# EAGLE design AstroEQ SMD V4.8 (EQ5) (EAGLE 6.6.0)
REVISION: V4.8
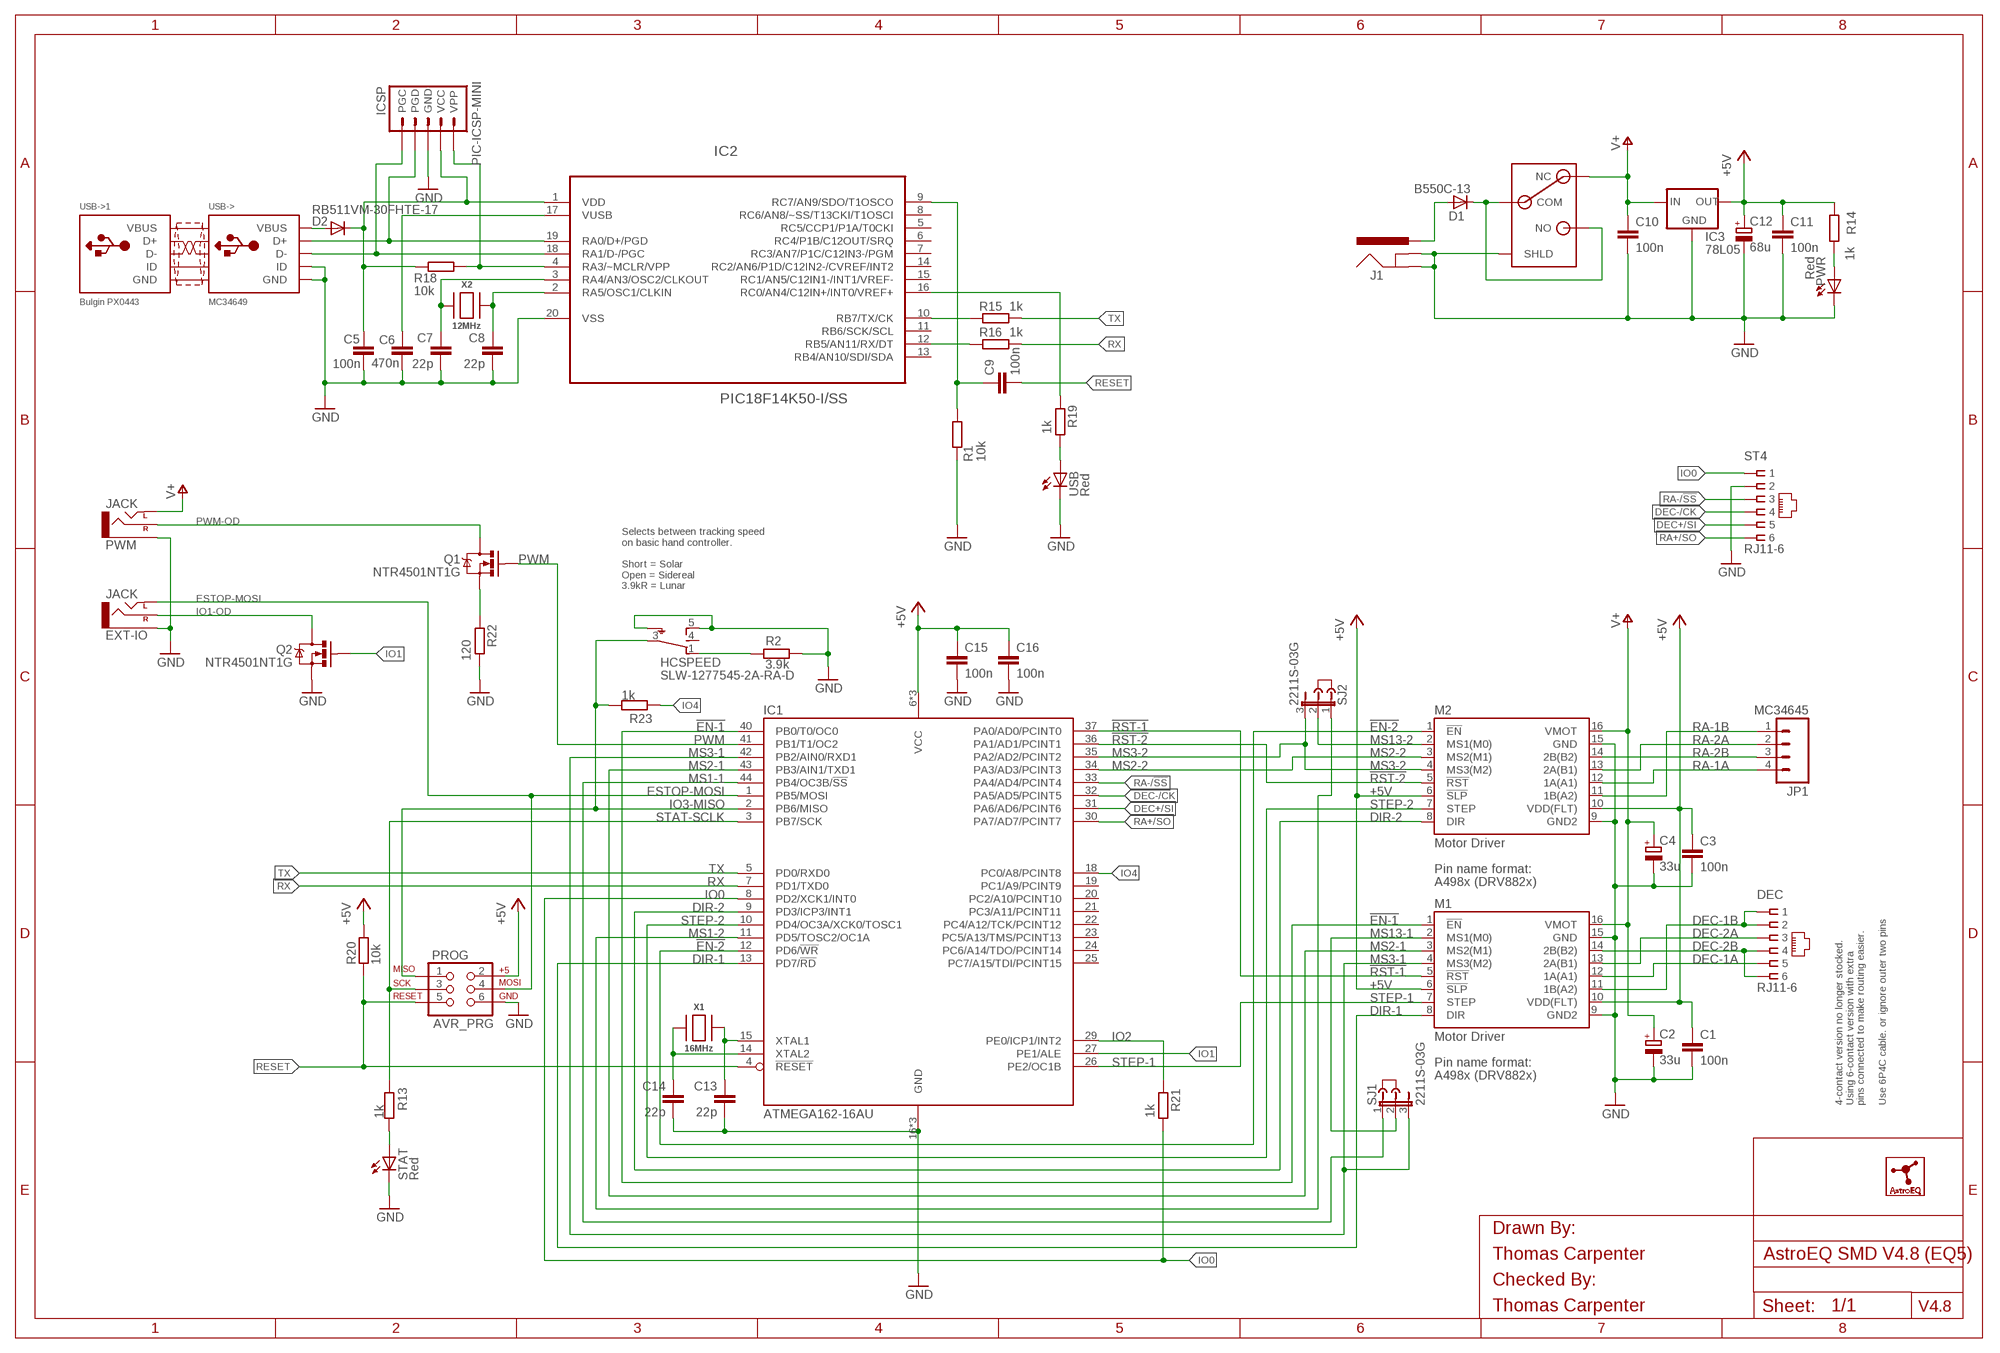
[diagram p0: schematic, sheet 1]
FRAME1 (A3L-LOC): CHECKED_BY: Thomas Carpenter; DRAWN_BY: Thomas Carpenter
USB->1 (USB-PANEL): MF: BULGIN; MPN: PX0443; OC_FARNELL: 1229685

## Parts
C1  100n  C-EUC0603  [C0603]
C2  33u  CPOL-EUSMCC  [SMC_C]
C3  100n  C-EUC0603  [C0603]
C4  33u  CPOL-EUSMCC  [SMC_C]
C5  100n  C-EUC0603  [C0603]
C6  470n  C-EUC0603  [C0603]
C7  22p  C-EUC0603  [C0603]
C8  22p  C-EUC0603  [C0603]
C9  100n  C-EUC0603  [C0603]
C10  100n  C-EUC0603  [C0603]
C11  100n  C-EUC0603  [C0603]
C12  68u  CPOL-EUSMCC  [SMC_C]
C13  22p  C-EUC0603  [C0603]
C14  22p  C-EUC0603  [C0603]
C15  100n  C-EUC0603  [C0603]
C16  100n  C-EUC0603  [C0603]
D1  B550C-13  DIODE-SMC  [SMC]
D2  RB511VM-30FHTE-17  DIODESOD  [SOD-323]
DEC  RJ11-6  RJ11-2L-B  [RJ11-NO_SHIELD]
EXT-IO  JACK  AUDIO-JACKVERT  [AUDIO-JACK-3.5MM-VERT]
HCSPEED  SLW-1277545-2A-RA-D  [SLW-127]
IC1  ATMEGA162-16AU  [TQFP44]
IC2  PIC18F14K50-I/SS  [SS20]
IC3  78L05  78LXXSOT-23  [SOT23]
ICSP  PIC-ICSP-MINI  [PIC-ICSP-MINI]
J1  POWER_JACKPANEL  [POWER_JACK_PANEL]
J2  DNI  JUMPER  [JUMP]
J3  DNI  JUMPER  [JUMP]
JP1  MC34645  M04POLAR  [MOLEX-1X4]
LOGO1  ASTROEQ5MM  [ASTROEQ-SMALL]
M1  Motor Driver  A4983CARRIER  [DIP16-W]
M2  Motor Driver  A4983CARRIER  [DIP16-W]
PROG  AVR_PRG  AVR_SPI_PRG_6PTH  [2X3]
PWM  JACK  AUDIO-JACKVERT  [AUDIO-JACK-3.5MM-VERT]
PWR  Red  LED3MM  [LED3MM]
PWR-SW  SWITCH  [SPST]
Q1  NTR4501NT1G  MOSFET-NCHANNELSMD  [SOT23-3]
Q2  NTR4501NT1G  MOSFET-NCHANNELSMD  [SOT23-3]
R1  10k  R-EU_R0603  [R0603]
R2  3.9k  R-EU_R0603  [R0603]
R13  1k  R-EU_R0603  [R0603]
R14  1k  R-EU_R0603  [R0603]
R15  1k  R-EU_R0603  [R0603]
R16  1k  R-EU_R0603  [R0603]
R18  10k  R-EU_R0603  [R0603]
R19  1k  R-EU_R0603  [R0603]
R20  10k  R-EU_R0603  [R0603]
R21  1k  R-EU_R0603  [R0603]
R22  120  R-EU_R0805  [R0805]
R23  1k  R-EU_R0603  [R0603]
SJ1  2211S-03G  JP2E  [JP2]
SJ2  2211S-03G  JP2E  [JP2]
ST4  RJ11-6  RJ11-2L-B  [RJ11-NO_SHIELD]
STAT  Red  LED3MM  [LED3MM]
USB  Red  LED3MM  [LED3MM]
USB->  MC34649  USBBULGINWIRE  [22-23-2051]
X1  16MHz  XTALNX5032  [NX5032]
X2  12MHz  XTALNX5032  [NX5032]

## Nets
!EN-1: IC1.40(PB0/T0/OC0) M1.1(!EN)
!EN-2: IC1.12(PD6/!WR) M2.1(!EN)
!RST-1: IC1.37(PA0/AD0/PCINT0) M1.5(!RST)
!RST-2: IC1.36(PA1/AD1/PCINT1) M2.5(!RST)
+5V: C1.1 C3.1 C11.1 C12.+ C15.1 C16.1 IC1.6(VCC) IC1.17(VCC) IC1.38(VCC) IC3.1(OUT) M1.6(!SLP) M1.10(VDD(FLT)) M2.6(!SLP) M2.10(VDD(FLT)) PROG.2 R14.1 R20.2
AVROSC1: C13.1 IC1.15(XTAL1) X1.1
AVROSC2: C14.1 IC1.14(XTAL2) X1.2
D_N [usbdat]: IC2.18(RA1/D-/PGC) ICSP.5(PGC) USB->.2(D-)
D_P [usbdat]: IC2.19(RA0/D+/PGD) ICSP.4(PGD) USB->.3(D+)
DEC+/SI: IC1.31(PA6/AD6/PCINT6) ST4.5
DEC-1A: DEC.5 M1.12(1A(A1))
DEC-1B: DEC.1 DEC.2 M1.11(1B(A2))
DEC-2A: DEC.3 M1.13(2A(B1))
DEC-2B: DEC.4 DEC.6 M1.14(2B(B2))
DEC-/CK: IC1.32(PA5/AD5/PCINT5) ST4.4
DIR-1: IC1.13(PD7/!RD) M1.8(DIR)
DIR-2: IC1.9(PD3/ICP3/INT1) M2.8(DIR)
DTR: C9.1 IC2.9(RC7/AN9/SDO/T1OSCO) R1.1
ESTOP-MOSI: EXT-IO.2(LEFT) IC1.1(PB5/MOSI) PROG.4
GND: C1.2 C2.- C3.2 C4.- C5.2 C6.1 C7.2 C8.2 C10.2 C11.2 C12.- C13.2 C14.2 C15.2 C16.2 EXT-IO.1(SLEEVE) HCSPEED.5(O) HCSPEED.S1(SH) HCSPEED.S2(SH) IC1.16(GND) IC1.28(GND) IC1.39(GND) IC2.20(VSS) IC3.3(GND) ICSP.3(GND) J1.SHUNT(GNDBREAK) J1.SLEEVE(GND) M1.9(GND2) M1.15(GND) M2.9(GND2) M2.15(GND) PROG.6 PWM.1(SLEEVE) PWR-SW.S1(SHLD) PWR-SW.S2(SHLD) PWR-SW.S3(SHLD) PWR-SW.S4(SHLD) PWR.K(C) Q2.2(S) R1.2 R2.2 R22.1 ST4.2 STAT.K(C) USB->.4(GND) USB->.5(ID) USB.K(C)
IO0: IC1.8(PD2/XCK1/INT0) R21.1 ST4.1
IO1: IC1.27(PE1/ALE) Q2.1(G)
IO1-OD: EXT-IO.3(RIGHT) Q2.3(D)
IO2: IC1.29(PE0/ICP1/INT2) R21.2
IO3-MISO: HCSPEED.3(P) IC1.2(PB6/MISO) PROG.1 R23.2
IO4: IC1.18(PC0/A8/PCINT8) R23.1
MCLR: IC2.4(RA3/~MCLR/VPP) ICSP.1(VPP) R18.1
MS1-1: IC1.44(PB4/OC3B/!SS) SJ1.1
MS1-2: IC1.11(PD5/TOSC2/OC1A) SJ2.1
MS2-1: IC1.43(PB3/AIN1/TXD1) M1.3(MS2(M1))
MS2-2: IC1.34(PA3/AD3/PCINT3) M2.3(MS2(M1))
MS3-1: IC1.42(PB2/AIN0/RXD1) M1.4(MS3(M2)) SJ1.3
MS3-2: IC1.35(PA2/AD2/PCINT2) M2.4(MS3(M2)) SJ2.3
MS13-1: M1.2(MS1(M0)) SJ1.2
MS13-2: M2.2(MS1(M0)) SJ2.2
N$1: HCSPEED.1(S) R2.1
PWM: IC1.41(PB1/T1/OC2) Q1.1(G)
PWM-OD: PWM.3(RIGHT) Q1.3(D)
PWM-RES: Q1.2(S) R22.2
PWRLED: PWR.A R14.2
RA+/SO: IC1.30(PA7/AD7/PCINT7) ST4.6
RA-1A: JP1.4 M2.12(1A(A1))
RA-1B: JP1.1 M2.11(1B(A2))
RA-2A: JP1.2 M2.13(2A(B1))
RA-2B: JP1.3 M2.14(2B(B2))
RA-/!SS: IC1.33(PA4/AD4/PCINT4) ST4.3
RESET: C9.2 IC1.4(!RESET) PROG.5 R20.1
RX: IC1.7(PD1/TXD0) R16.1
RX(USB): IC2.12(RB5/AN11/RX/DT) R16.2
STAT-SCLK: IC1.3(PB7/SCK) PROG.3 R13.1
STATLED: R13.2 STAT.A
STEP-1: IC1.26(PE2/OC1B) M1.7(STEP)
STEP-2: IC1.10(PD4/OC3A/XCK0/TOSC1) M2.7(STEP)
SWITCH: D1.C PWR-SW.COM PWR-SW.NO
TX: IC1.5(PD0/RXD0) R15.1
TX(USB): IC2.10(RB7/TX/CK) R15.2
USBLED: R19.1 USB.A
USBOSC1: C8.1 IC2.2(RA5/OSC1/CLKIN) X2.2
USBOSC2: C7.1 IC2.3(RA4/AN3/OSC2/CLKOUT) X2.1
USBSTAT: IC2.16(RC0/AN4/C12IN+/INT0/VREF+) R19.2
V+: C2.+ C4.+ C10.1 IC3.2(IN) M1.16(VMOT) M2.16(VMOT) PWM.2(LEFT) PWR-SW.NC
VBUS: D2.2(A) USB->.1(VBUS)
VIN: D1.A J1.CENTRE(PWR)
VPIC: C5.1 D2.1(C) IC2.1(VDD) ICSP.2(VCC) R18.2
VUSB: C6.2 IC2.17(VUSB)
Unconnected: HCSPEED.4(M) IC1.19(PC1/A9/PCINT9) IC1.20(PC2/A10/PCINT10) IC1.21(PC3/A11/PCINT11) IC1.22(PC4/A12/TCK/PCINT12) IC1.23(PC5/A13/TMS/PCINT13) IC1.24(PC6/A14/TDO/PCINT14) IC1.25(PC7/A15/TDI/PCINT15) IC2.5(RC5/CCP1/P1A/T0CKI) IC2.6(RC4/P1B/C12OUT/SRQ) IC2.7(RC3/AN7/P1C/C12IN3-/PGM) IC2.8(RC6/AN8/~SS/T13CKI/T1OSCI) IC2.11(RB6/SCK/SCL) IC2.13(RB4/AN10/SDI/SDA) IC2.14(RC2/AN6/P1D/C12IN2-/CVREF/INT2) IC2.15(RC1/AN5/C12IN1-/INT1/VREF-)

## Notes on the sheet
- Selects between tracking speed
  on basic hand controller.
  
  Short = Solar
  Open = Sidereal
  3.9kR = Lunar
- 4-contact version no longer stocked.
  Using 6-contact version with extra
  pins connected to make routing easier.
  
  Use 6P4C cable. or ignore outer two pins

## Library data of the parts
C1 C3 C5 C9-C11 C15 C16 = rcl:C-EU: CAPACITOR, European symbol; MF: MULTICOMP; MPN: MC0603F104Z250CT; OC_FARNELL: 1759038
C2 C4 = rcl:CPOL-EU: POLARIZED CAPACITOR, European symbol; MF: KEMET; MPN: T491C336K025AT; OC_FARNELL: 1793896
C6 = rcl:C-EU: CAPACITOR, European symbol; MF: MULTICOMP; MPN: MC0603F474Z160CT; OC_FARNELL: 1759021
C7 C8 C13 C14 = rcl:C-EU: CAPACITOR, European symbol; MF: MULTICOMP; MPN: MC0603N220J500CT; OC_FARNELL: 1759057
C12 = rcl:CPOL-EU: POLARIZED CAPACITOR, European symbol; MF: AVX; MPN: TPSC686K016R0125; OC_FARNELL: 1658976
D1 = diode:DIODE-: DIODE; MF: DIODES INC.; MPN: B550C-13-F; OC_FARNELL: 1858608
D2 = SparkFun:DIODE: Diode; MF: ROHM; MPN: RB511VM-30FHTE-17; OC_FARNELL: 2581544
DEC ST4 = con-tycoelectronics:RJ11: CORCOM Modular RJ Jacks No Shield Source: www.tycoelectronics.com .. ENG_DS_1654001_1099_RJ_L_0507.pdf; MF: MOLEX; MPN: 95503-2661; OC_FARNELL: 1620210
EXT-IO PWM = SparkFun:AUDIO-JACK: 3.5mm Audio Jack Simple 3.5mm common PCB mount audio jack. SKU: PRT-08032; MANUFACTURER: LUMBERG; MF: LUMBERG; MPN: 1502 01; OC_FARNELL: 1243242
HCSPEED = switch:SLW-127
IC1 = atmel:ATMEGA162: 8-bit RISC MICROCONTROLLER 16K Bytes internal flash program memory 1K Bytes internal SRAM Upto 64K Bytes optional external memory space 512 Bytes EEPROM Two 8-bit timers Two 16-bit timers Dual programmable serial USARTs Master/Slave serial SPI interface Source: ATMEGA162_DIP40.lbr; MF: ATMEL; MPN: ATMEGA162-16AU; OC_FARNELL: 9171150
IC2 = microchip:PIC18F14K50: USB Flash Microcontrollers; MF: MICROCHIP
IC3 = v-reg:78LXX: VOLTAGE REGULATOR; MF: TAIWAN SEMICONDUCTOR; MPN: TS78L05CX RFG; OC_FARNELL: 1476698
ICSP = SparkFun:PIC-ICSP-MINI: PIC-ICSP-Mini Miniature 5-pin connection for temporary programming of PICs. Use this device in your design to save space. Program the PIC with this adapter Spark Fun Electronics SKU : BOB-00194; OC_FARNELL: unknown
J1 = SparkFun:POWER_JACK: Power Jack This is the standard 5.5mm barrel jack for power. The PTH is the most common, proven, reliable, footprint. All others are experimental. The Slot footprint only works if the mill layer is transmitted to the PCB fab house so be warned. Spark Fun Electronics SKU : PRT-00119. Mating wall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; MF: SWITCHCRAFT; MPN: PCL712AS; OC_FARNELL: 1871167
J2 J3 = jumper:JUMPER: JUMPER header; MF: 3M; MPN: 969102-0000-DA; OC_FARNELL: 2579814
JP1 = SparkFun:M04: Header 4 Standard 4-pin 0.1" header. Use with straight break away headers (SKU : PRT-00116), right angle break away headers (PRT-00553), swiss pins (PRT-00743), machine pins (PRT-00117), and female headers (PRT-00115). Molex polarized connector foot print use with SKU : PRT-08231 with associated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; MF: MULTICOMP; MPN: MC34645; OC_FARNELL: 1675775
LOGO1 = AstroEQTooth:ASTROEQ; OC_FARNELL: unknown
M1 M2 = A4983Carrier:A4983CARRIER; MF: SAMTEC; MPN: CES-116-01-T-S; OC_FARNELL: 1667522
PROG = SparkFun:AVR_SPI_PRG_6: AVR ISP 6 Pin This is the reduced ISP connector for AVR programming. Common on Arduino. This footprint will take up less PCB space and can be used with a 10-pin to 6-pin adapter such as SKU: BOB-08508; MF: AMP - TE CONNECTIVITY; MPN: 826632-3; OC_FARNELL: 3418492
PWR STAT USB = led:LED: LED; MF: KINGBRIGHT; MPN: L-424HDT; OC_FARNELL: 1142499
PWR-SW = con-tycoelectronics:SWITCH; MF: TE CONNECTIVITY; MPN: AE101J1V3B004; OC_FARNELL: 1813654
Q1 Q2 = SparkFun:MOSFET-NCHANNEL; MF: ON SEMICONDUCTOR; MPN: NTR4501NT1G; OC_FARNELL: 1431305
R1 R18 R20 = rcl:R-EU_: RESISTOR, European symbol; MF: MULTICOMP; MPN: MCWR06X1002FTL; OC_FARNELL: 2447230
R2 R13-R16 R19 R21 R23 = rcl:R-EU_: RESISTOR, European symbol; MF: MULTICOMP; MPN: MCWR06X1001FTL; OC_FARNELL: 2447272
R22 = rcl:R-EU_: RESISTOR, European symbol; MF: MULTICOMP; MPN: MCWR08X1200FTL; OC_FARNELL: 2447561
SJ1 SJ2 = jumper:JP2E: JUMPER; MF: MULTICOMP; MPN: 2211S-03G; OC_FARNELL: 1593412
USB-> = adafruit:USB: USB Connectors USBMINIB - Surface Mount Female Mini-B USB Connector 4UConnector: 06564 By microbuilder.eu Thru-hole RA Female Mini-B USB Connector 4UConnector: 18732 By ladyada.net; MF: MULTICOMP; MPN: MC34647; OC_FARNELL: 1675776
X1 = adafruit:XTAL: Low cost SMT crystals, no capacitors included; MF: TXC; MPN: 7A-16.000MAAJ-T; OC_FARNELL: 1841946
X2 = adafruit:XTAL: Low cost SMT crystals, no capacitors included; MF: TXC; MPN: 7A-12.000MAAJ-T; OC_FARNELL: 1841940

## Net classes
1 power: width 0.61 mm, drill 0.711 mm, clearance 0.203 mm
2 gnd: width 0.305 mm, drill 0.711 mm, clearance 0.203 mm
3 usbvcc: width 0.508 mm, drill 0.711 mm, clearance 0.203 mm
4 usbdat: width 0.406 mm, clearance 0.152 mm

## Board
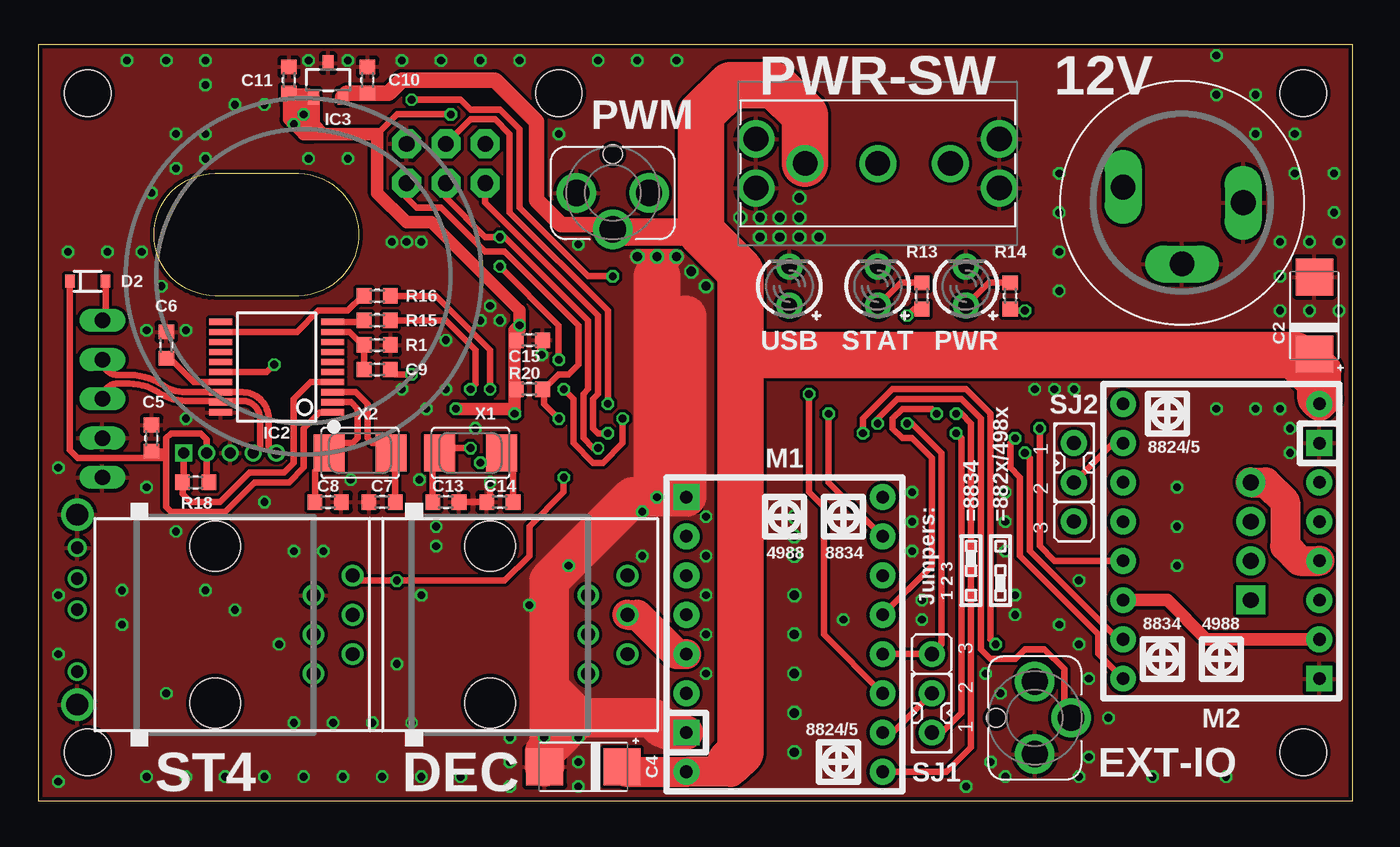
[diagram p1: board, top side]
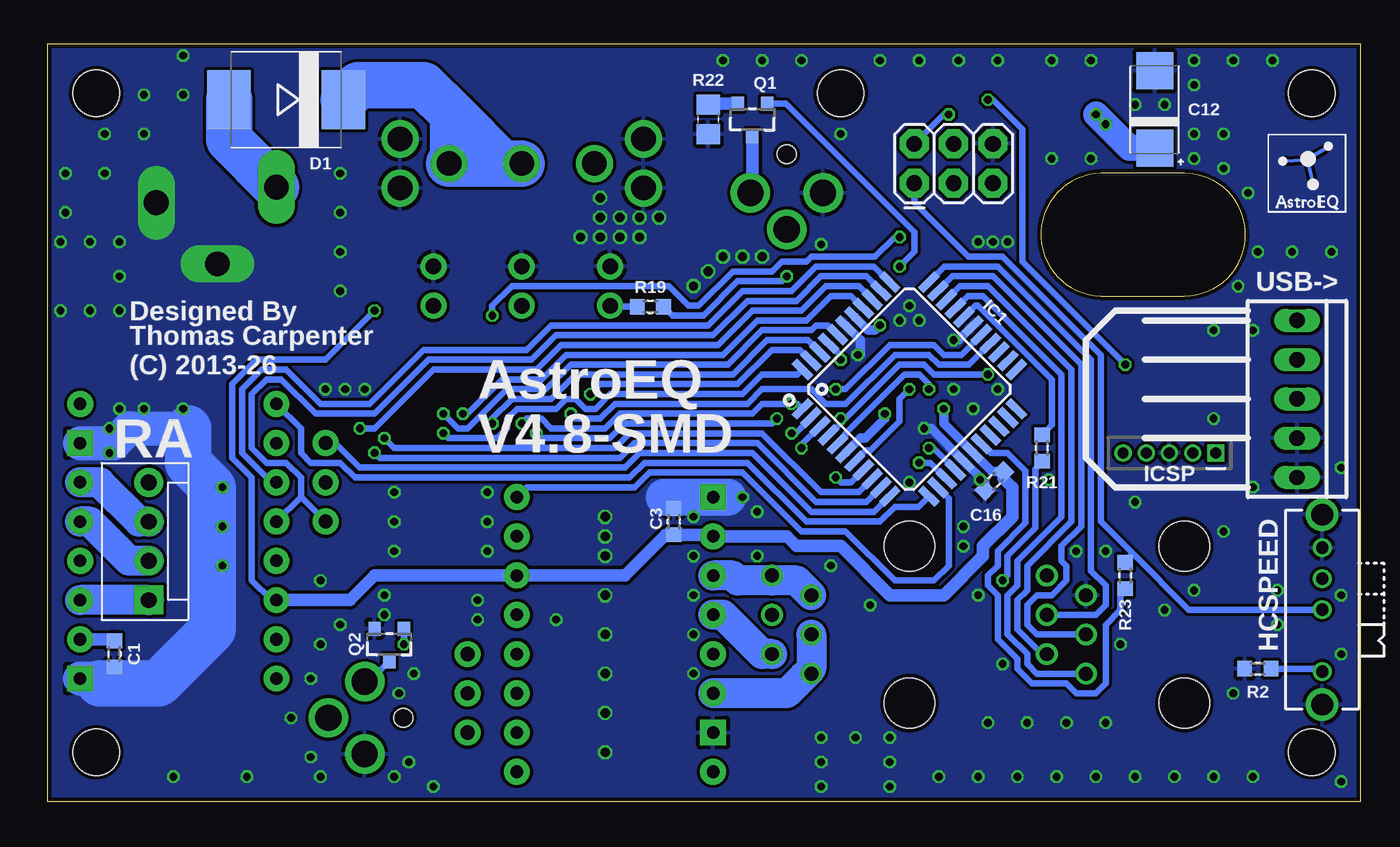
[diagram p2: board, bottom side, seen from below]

Size 85 x 49 mm. Coordinates in mm from the lower left corner, seen from the top.
Outline: 0,0 0,49 85,49 85,0 0,0
Outline: 16.83,40.64 arc-177 16.83,32.7 11.43,32.7 arc-180 11.43,40.64 16.83,40.64
Copper layers (1*16): Top 0.035mm / dielectric 1.5mm / Bottom 0.035mm
Design rules "ITEADstudio_DRC *": minimum track width 6mil, minimum drill 12mil, track to track 6mil, track to pad 6mil, pad to pad 6mil, via to via 6mil, smd to smd 0mil, copper to edge 10mil, drill to drill 10mil, minimum pad ring 8mil, minimum via ring 6mil, stop-mask expansion 2mil, vias tented up to drill 1mm, thermal gap 10mil
Holes 3 mm at 81.83,3.17 33.66,45.83 3.17,45.83 81.83,45.83 3.17,3.17
bKeepout: area 48.3,7.4 to 53.3,12.4

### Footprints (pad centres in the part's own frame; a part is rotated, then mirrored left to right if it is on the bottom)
C0603 = smd 0.95 x 1: 1 -0.85,0; 2 0.85,0
SMC_C = smd 2.4 x 2.4: + -2.5,0; - 2.5,0
SMC = smd 2.8 x 3.8: A 3.7,0; C -3.7,0
SOD-323 = smd 0.63 x 0.83: 1 -1.15,0; 2 1.15,0
RJ11-NO_SHIELD = drill 0.9 pad 1.4: 1 -3.175,8.89; 2 -1.905,6.35; 3 -0.635,8.89; 4 0.635,6.35; 5 1.905,8.89; 6 3.175,6.35 | hole 3.251: -5.08,0; 5.08,0
AUDIO-JACK-3.5MM-VERT = drill 1.7: 1 2.35,0; 2 0,2.35; 3 -2.35,0 | hole 1.2: 0,-2.5
SLW-127 = drill 0.8: 1 -4,0; 3 0,0; 4 2,0; 5 4,0 | drill 1.4: S1 -6.15,0; S2 6.15,0
TQFP44 = smd 1.5 x 0.5: 1 -5.8,4; 2 -5.8,3.2; 3 -5.8,2.4; 4 -5.8,1.6; 5 -5.8,0.8; 6 -5.8,0; 7 -5.8,-0.8; 8 -5.8,-1.6; 9 -5.8,-2.4; 10 -5.8,-3.2; 11 -5.8,-4; 23 5.8,-4; 24 5.8,-3.2; 25 5.8,-2.4; 26 5.8,-1.6; 27 5.8,-0.8; 28 5.8,0; 29 5.8,0.8; 30 5.8,1.6; 31 5.8,2.4; 32 5.8,3.2; 33 5.8,4 | smd 0.5 x 1.5: 12 -4,-5.8; 13 -3.2,-5.8; 14 -2.4,-5.8; 15 -1.6,-5.8; 16 -0.8,-5.8; 17 0,-5.8; 18 0.8,-5.8; 19 1.6,-5.8; 20 2.4,-5.8; 21 3.2,-5.8; 22 4,-5.8; 34 4,5.8; 35 3.2,5.8; 36 2.4,5.8; 37 1.6,5.8; 38 0.8,5.8; 39 0,5.8; 40 -0.8,5.8; 41 -1.6,5.8; 42 -2.4,5.8; 43 -3.2,5.8; 44 -4,5.8
SS20 = smd 0.4 x 1.5: 1 -2.925,-3.625; 2 -2.275,-3.625; 3 -1.625,-3.625; 4 -0.975,-3.625; 5 -0.325,-3.625; 6 0.325,-3.625; 7 0.975,-3.625; 8 1.625,-3.625; 9 2.275,-3.625; 10 2.925,-3.625; 11 2.925,3.625; 12 2.275,3.625; 13 1.625,3.625; 14 0.975,3.625; 15 0.325,3.625; 16 -0.325,3.625; 17 -0.975,3.625; 18 -1.625,3.625; 19 -2.275,3.625; 20 -2.925,3.625
SOT23 = smd 0.7 x 1: 1 -0.95,-1.1; 2 0.95,-1.1; 3 0,1.1
PIC-ICSP-MINI = drill 0.7 square: 1 -3,0 | drill 0.7: 2 -1.5,0; 3 0,0; 4 1.5,0; 5 3,0
POWER_JACK_PANEL = drill 1.6 long: CENTRE 3.81,-1.016; SHUNT -3.962,0; SLEEVE 0,3.962
MOLEX-1X4 = drill 1.016 pad 1.88 square: 1 0,0 | drill 1.016 pad 1.88: 2 2.54,0; 3 5.08,0; 4 7.62,0
DIP16-W = drill 0.813 pad 1.676: 1 -8.89,-6.35; 2 -6.35,-6.35; 3 -3.81,-6.35; 4 -1.27,-6.35; 5 1.27,-6.35; 6 3.81,-6.35; 7 6.35,-6.35; 8 8.89,-6.35; 10 6.35,6.35; 11 3.81,6.35; 12 1.27,6.35; 13 -1.27,6.35; 14 -3.81,6.35; 16 -8.89,6.35 | drill 0.813 pad 1.676 square: 9 8.89,6.35; 15 -6.35,6.35
2X3 = drill 1.016 pad 1.88 octagon: 1 -2.54,-1.27; 2 -2.54,1.27; 3 0,-1.27; 4 0,1.27; 5 2.54,-1.27; 6 2.54,1.27
LED3MM = drill 1 pad 1.676: A -1.27,0; K 1.27,0
SPST = drill 1.6: COM 0,0; NC -4.699,0; NO 4.699,0; S1 7.874,1.587; S2 7.874,-1.587; S3 -7.874,1.587; S4 -7.874,-1.587
SOT23-3 = smd 0.8 x 0.9: 1 -0.95,-1; 2 0.95,-1; 3 0,1.1
R0603 = smd 0.95 x 1: 1 -0.85,0; 2 0.85,0
R0805 = smd 1.3 x 1.5: 1 -0.95,0; 2 0.95,0
JP2 = drill 0.914 pad 1.676: 1 -2.54,0; 2 0,0; 3 2.54,0
22-23-2051 = drill 1 long: 1 -5.08,0; 2 -2.54,0; 3 0,0; 4 2.54,0; 5 5.08,0
NX5032 = smd 2 x 2.4: 1 2,0; 2 -2,0

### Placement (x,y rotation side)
C1  80.64,9.53 270 bottom
C2  82.55,31.43 90 top
C3  44.45,18.1 90 bottom
C4  35.24,2.22 180 top
C5  7.3,23.5 90 top
C6  8.26,29.53 270 top
C7  22.23,19.37 180 top
C8  18.73,19.37 0 top
C9  21.91,27.94 0 top
C10  21.27,46.67 90 top
C11  16.19,46.67 90 top
C12  13.34,44.77 90 bottom
C13  26.35,19.37 0 top
C14  29.84,19.37 180 top
C15  31.75,29.84 0 top
C16  23.72,20.73 225 bottom
D1  69.53,45.4 180 bottom
D2  3.17,33.66 0 top
DEC  29.21,11.43 270 top
EXT-IO  64.45,5.4 270 top
HCSPEED  2.5,12.4 90 bottom
IC1  29.21,26.67 45 bottom
IC2  15.4,28.1 90 top
IC3  18.73,46.67 0 top
ICSP  12.38,22.54 180 bottom
J1  73.98,38.73 180 top
J2  57.78,5.71 0 top
J3  66.99,21.91 0 top
JP1  78.42,13.02 90 bottom
LOGO1  6.03,38.1 0 bottom
M1  48.26,10.79 90 top
M2  76.52,16.83 270 top
PROG  26.35,41.27 0 bottom
PWM  37.15,39.37 180 top
PWR  60.01,33.34 90 top
PWR-SW  54.29,41.27 0 top
Q1  39.37,44.13 180 bottom
Q2  62.87,10.16 180 bottom
R1  21.91,29.53 0 top
R2  6.67,8.57 180 bottom
R13  57.15,32.7 90 top
R14  62.87,32.7 90 top
R15  21.91,31.11 180 top
R16  21.91,32.7 180 top
R18  10.16,20.64 0 top
R19  45.97,32 0 bottom
R20  31.75,26.67 180 top
R21  20.64,22.86 90 bottom
R22  42.23,44.13 90 bottom
R23  15.24,14.61 90 bottom
SJ1  57.78,6.99 90 top
SJ2  66.99,20.64 270 top
ST4  11.43,11.43 270 top
STAT  54.29,33.34 90 top
USB  48.58,33.34 90 top
USB->  4.13,26.04 270 bottom
X1  27.94,22.54 180 top
X2  20.8,22.54 0 top

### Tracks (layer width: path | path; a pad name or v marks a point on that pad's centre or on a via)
!EN-1  (via drill 0.5)
  Top 0.406: M1.1 58.74,1.91 60.33,3.49 60.33,24.45 59.69,25.08 v59.37,25.08
  Bottom 0.406: IC1.40 34.47,30.8 35.24,30.8 35.56,30.48 38.73,30.48 40.96,28.26 51.12,28.26 52.7,26.67 55.24,26.67 57.78,24.13 58.42,24.13 v59.37,25.08
!EN-2
  Bottom 0.406: IC1.12 28.63,19.05 30.16,19.05 31.11,18.1 35.88,18.1 39.69,21.91 46.35,21.91 47.31,20.95 65.09,20.95 66.04,21.91 67.94,21.91 68.58,22.54 68.58,24.13 M2.1
!RST-1  (via drill 0.5)
  Top 0.406: M1.5 57.78,15.24 57.78,22.23 56.52,23.5 55.88,23.5 55.24,24.13 55.24,24.77 55.88,25.4 57.78,25.4 v58.1,25.08
  Bottom 0.406: IC1.37 32.98,32.7 34.29,32.7 35.88,31.11 39.05,31.11 41.27,28.89 51.44,28.89 53.02,27.3 55.56,27.3 57.78,25.08 v58.1,25.08
!RST-2  (via drill 0.5)
  Top 0.406: M2.5 65.72,15.56 64.77,16.51 v64.77,24.13
  Bottom 0.406: IC1.36 32.48,33.34 34.61,33.34 36.2,31.75 39.37,31.75 41.59,29.53 51.75,29.53 53.34,27.94 60.01,27.94 63.82,24.13 v64.77,24.13
+5V  (via drill 0.5)
  Top 0.406: 31.11,30.48 30.8,30.48 | v26.67,44.45 23.18,44.45 21.91,43.18 | R14.1 62.97,31.75 v63.82,31.75
  Top 0.813: R20.2 30.8,26.67 | v26.99,25.4 30.8,25.4 | 30.8,25.4 v30.8,25.08 | 30.8,29.84 30.8,26.67 | 30.8,26.67 30.8,25.4 | v31.11,30.8 30.8,30.48 30.8,29.84 | 30.8,29.84 C15.1 | v31.11,30.8 31.11,31.75 25.4,37.47 23.81,37.47 21.91,39.37 21.91,43.18 18.41,43.18 | v31.11,30.8 31.11,30.48 | M2.6 73.03,13.02 75.56,10.48 M2.10 | 18.41,43.18 17.78,43.81 | 17.78,43.81 IC3.1 | 16.19,45.4 C11.1 16.41,45.82 16.51,45.72 | 16.19,45.4 16.83,44.77 16.83,44.45 16.19,45.09 | 16.19,45.09 16.19,45.4 | 16.19,45.09 16.19,44.13 v16.51,43.81 17.14,43.18 17.78,43.18 | 18.41,43.18 17.78,43.18 | 17.78,43.18 17.14,43.81 v17.14,44.45 17.78,43.81 | 16.51,45.72 17.78,44.45 17.78,45.4 17.46,45.72 16.51,45.72
  Bottom 0.406: PROG.2 26.99,44.45 v26.67,44.45 | v63.82,31.75 66.99,28.57 71.44,28.57 73.03,26.99 73.03,22.23 71.75,20.95 71.75,14.29 70.48,13.02 M2.6
  Bottom 0.61: C16.1 23.87,21.33 IC1.17 26.99,24.45 v26.99,25.4 | v30.8,25.08 30.8,24.77 32.07,23.5 32.38,23.5 IC1.6 | IC1.38 31.89,30.48 31.43,30.48 v31.11,30.8
  Bottom 0.813: C16.1 23.12,20.9 22.54,20.32 22.54,18.41 24.45,16.51 24.45,15.88 26.99,13.34 30.48,13.34 33.66,16.51 36.51,16.51 37.15,17.14 M1.10 42.01,17.25 C3.1 44.98,17.25 47.62,14.61 M1.6 63.82,14.61 65.41,13.02 M2.6 | 80.54,10.48 C1.1 80.75,10.48 M2.10
  Bottom 1.676: C12.+ 14.96,42.27 v17.14,44.45
AVROSC1  (via drill 0.5)
  Top 0.406: v27.94,22.86 26.26,22.86 X1.1 25.5,22.11 C13.1
  Bottom 0.406: IC1.15 27.66,22.86 v27.94,22.86
AVROSC2  (via drill 0.5)
  Top 0.406: v28.57,21.91 29.3,21.91 X1.2 30.7,21.79 C14.1
  Bottom 0.406: IC1.14 27.84,21.91 v28.57,21.91
D_N
  Top 0.406: USB->.2 arc90 5.12,27.58 5.87,27.58 arc-34 8.1,26.9 arc35 9.52,26.47 IC2.18 | ICSP.5 arc-90 14.88,23.04 14.88,24.77 arc90 13.18,26.47 IC2.18 | IC2.18
D_P
  Top 0.406: USB->.3 arc-90 5.12,27.03 5.87,27.03 arc-34 7.78,26.44 arc35 9.53,25.91 11.77,25.91 | ICSP.4 arc90 14.33,22.99 14.33,24.77 arc90 13.18,25.91 11.77,25.91 | IC2.19 11.77,25.91
DEC+/SI
  Bottom 0.406: IC1.31 25.94,33.34 24.13,33.34 18.73,27.94 18.73,18.1 21.59,15.24 21.59,13.65 22.23,13.02 22.23,11.11 20.64,9.53 ST4.5
DEC-1A
  Bottom 1.93: DEC.5 38.73,9.53 41.27,12.06 M1.12
DEC-1B
  Bottom 0.406: DEC.1 38.1,14.29
  Bottom 1.93: DEC.2 36.51,14.29 38.1,14.29 40.32,14.29 40.64,14.61 M1.11
DEC-2A
  Top 1.93: DEC.3 38.73,12.06 41.27,9.53 M1.13
DEC-2B
  Bottom 0.406: DEC.6 36.04,8.26 36.04,8.1
  Bottom 1.93: DEC.4 35.56,8.57 36.04,8.1 37.15,6.99 M1.14
DEC-/CK
  Bottom 0.406: IC1.32 26.43,33.97 23.81,33.97 18.1,28.26 18.1,17.78 19.37,16.51 19.37,15.56 19.05,15.24 19.05,14.29 20,13.34 20.95,13.34 21.59,12.7 21.59,11.43 20.95,10.79 ST4.4
DIR-1
  Bottom 0.406: IC1.13 26.67,19.61 26.67,15.24 27.62,14.29 30.16,14.29 33.34,17.46 36.2,17.46 40.01,21.27 46.04,21.27 46.99,20.32 53.98,20.32 M1.8
DIR-2  (via drill 0.5)
  Top 0.406: M2.8 68.58,9.53 68.58,10.79 63.5,15.88 63.5,20.95 62.87,21.59 62.87,23.18 v63.18,23.5
  Bottom 0.406: IC1.9 32.48,20 34.92,20 38.73,23.81 47.31,23.81 48.26,22.86 62.55,22.86 v63.18,23.5
DTR
  Top 0.406: IC2.9 20.11,30.37 20.95,29.53 R1.1 C9.1
ESTOP-MOSI  (via drill 0.5)
  Top 0.406: v36.83,25.72 36.83,31.75 30.48,38.1 30.48,43.18 29.53,44.13 27.94,44.13 PROG.4 | v54.29,24.45 54.29,24.77 55.56,26.04 59.69,26.04 60.96,24.77 60.96,9.84 61.59,9.21 63.18,9.21 63.82,9.84 65.09,9.84 66.36,8.57 66.36,5.84 EXT-IO.2
  Bottom 0.406: IC1.1 36.46,25.72 v36.83,25.72 38.73,25.72 39.37,25.08 47.94,25.08 48.9,24.13 52.39,24.13 53.02,24.77 53.98,24.77 v54.29,24.45
GND  (via drill 0.5, 0.6)
  Top 0.406: C13.2 C14.2 29.21,19.58 v29.21,20.64
  Top 0.61: C15.2 32.54,29.84 v32.54,28.89
  Top 1.016: v38.73,35.24 v40.01,35.24 v41.27,35.24 40.01,33.97
  Top 2.184: 40.32,4.76 40.64,4.45 M1.15
  Top 2.54: C4.- 32.74,3.21 33.02,3.49 | 33.02,3.49 34.92,5.4 | 34.92,5.4 39.69,5.4 40.32,4.76 | 34.92,5.4 33.02,7.3 | 33.02,7.3 33.02,14.29 38.42,19.68 M1.9 41.91,31.43 40.01,31.43 | 33.02,7.3 33.02,3.49
  Top 3: 40.01,20.32 40.01,31.43 40.01,33.97
  Bottom 0.61: C16.2 24.32,20.65 IC1.16 27.8,24.13 v28.26,24.13 | IC1.28 26.04,29.84 | IC1.39 32.38,29.84 32.38,28.89 v32.54,28.89
  Bottom 0.813: C1.2 81.38,7.94
  Bottom 2.184: 81.38,7.94 M2.9 | M2.15 80.64,23.18 79.69,24.13 75.88,24.13
  Bottom 2.4: 45.09,19.68 40.96,19.68
  Bottom 3: 75.88,24.13 75.88,21.91 74.3,20.32 74.3,11.11 77.79,7.62 81.6,7.62
  other vias: 14.61,19.37 16.51,16.19 26.35,29.84 25.72,17.78 9.53,24.77 9.53,30.48 25.72,16.51 47.94,36.51 43.18,33.34 49.21,39.05 23.5,26.67 28.57,31.11 29.84,31.11 25.08,25.4 26.35,26.67 50.48,36.51 46.67,36.51 22.86,36.2 29.21,32.07 49.21,36.51 47.94,37.78 49.21,37.78 45.4,37.78 46.67,37.78 42.23,34.29 48.9,3.17 48.9,5.71 48.9,8.26 48.9,10.79 48.9,13.34 48.9,15.88 48.9,18.41 23.18,8.89 24.77,13.34 34.29,15.24 39.05,18.73 30.48,0.95 30.48,4.13 34.92,4.13 34.92,0.95 32.7,4.13 30.48,2.54 34.92,2.54 43.18,8.26 43.18,10.79 43.18,13.34 43.18,15.88 39.05,15.88 23.81,36.2 24.77,36.2 34.92,36.04 84.14,36.2 84.14,31.75 82.23,36.2 80.33,36.2 80.33,33.97 80.33,31.75 82.23,31.75 10.79,47.94 10.79,46.35 12.7,45.09 14.61,45.09 17.46,47.94 20,47.94 23.5,47.94 26.04,47.94 28.57,47.94 31.11,47.94 36.2,47.94 38.73,47.94 41.27,47.94 33.66,43.18 7.94,33.34 8.89,40.96 8.89,43.18 10.79,43.18 20,41.59 1.27,21.59 8.26,6.99 1.27,9.53 1.27,13.34 1.27,1.27 22.23,1.59 19.68,1.59 17.14,1.59 14.61,1.59 12.06,1.59 9.53,1.59 6.99,1.59 24.77,1.59 27.3,1.59 62.23,6.99 67.31,10.16 76.83,1.59 61.59,2.54 73.66,15.24 73.66,17.78 73.66,20.32 76.2,25.4 78.74,25.4 66.04,33.02 66.04,35.56 78.74,45.72 81.28,43.18 83.82,40.64 81.28,40.64 78.74,43.18 76.2,48.26 76.2,45.72 83.82,38.1 6.99,30.48 6.99,20.32 8.89,17.46 5.4,13.65 1.91,35.56 4.45,35.56 6.67,35.56 17.46,41.59 10.79,41.59 7.3,39.37 8.26,47.94 5.71,47.94 31.75,12.7 16.51,5.08 19.05,5.08 21.59,5.08 24.13,5.08 63.18,12.06 57.15,11.75 67.31,14.29 52.07,11.75 56.52,20 56.52,16.19 66.04,38.1 66.04,40.64 12.7,12.38 63.18,13.34 60.01,0.95 62.55,1.59 67.31,1.59 72.07,1.59 48.9,17.14 40.01,19.68 43.18,18.41 80.96,24.13 80.96,22.54 80.33,25.4 64.45,26.67 66.99,26.67 65.72,26.67 62.55,20 62.55,18.1 62.55,16.19 66.04,11.43 67.94,7.94 69.22,5.4 67.94,2.86 61.28,8.26 57.15,13.02 56.52,18.1 10.79,13.65 5.4,11.43 18.41,16.19 24.63,20.81 20.18,20.81 15.56,10.16
  pour Bottom (isolate 0.203): -2.54,50.8 86.36,50.8 86.36,-2.54 -2.54,-2.54
  pour Top (isolate 0.203): -2.54,50.8 86.36,50.8 86.36,-2.54 -2.54,-2.54
  pour Bottom (isolate 0.203, no thermals): 78.74,43.18 76.2,43.18 71.12,38.1 71.12,33.02 81.28,33.02 81.28,40.64
IO0  (via drill 0.5)
  Top 0.406: ST4.1 20.64,14.29 v23.18,14.29 30.16,14.29 31.75,15.88 31.75,17.78 33.97,20 v33.97,20.95
  Bottom 0.406: R21.1 20.64,21.91 21.05,21.49 21.05,17.68 22.86,15.88 22.86,14.61 v23.18,14.29 | v33.97,20.95 33.66,20.64 32.98,20.64 IC1.8
IO1  (via drill 0.5)
  Top 0.406: v33.97,26.67 34.61,26.04 34.61,23.18 35.88,21.91 36.51,21.91 37.78,23.18 v37.78,24.77 | v53.34,23.81 53.34,24.77 55.24,26.67 60.01,26.67 61.59,25.08 61.59,10.48 v61.91,10.16
  Bottom 0.406: IC1.27 25.86,28.89 26.99,28.89 27.62,29.53 30.48,29.53 33.34,26.67 v33.97,26.67 | v37.78,24.77 38.1,24.45 47.62,24.45 48.58,23.5 53.02,23.5 v53.34,23.81 | v61.91,10.16 Q2.1
IO1-OD
  Bottom 0.406: Q2.3 64.18,7.75 EXT-IO.3
IO2
  Bottom 0.406: IC1.29 24.94,32.07 24.77,32.07 20,27.3 20,24.34 R21.2
IO3-MISO  (via drill 0.5)
  Top 0.406: v36.83,23.81 36.2,23.81 35.88,24.13 35.88,26.04 36.2,26.35 36.2,31.43 28.89,38.73 PROG.1
  Bottom 0.406: IC1.2 36.59,23.81 v36.83,23.81 | PROG.1 28.89,38.73 25.4,35.24 23.18,35.24 16.83,28.89 16.83,18.1 14.76,16.03 | 14.76,16.03 11.13,12.4 HCSPEED.3 | R23.2 15.24,15.56 14.76,16.03
IO4
  Bottom 0.406: R23.1 15.24,13.65 15.56,13.34 15.56,12.38 16.51,11.43 16.51,7.62 17.14,6.99 18.41,6.99 19.05,7.62 21.27,7.62 22.23,8.57 22.23,9.21 23.5,10.48 23.5,13.34 24.13,13.97 24.13,14.61 23.5,15.24 23.5,16.19 21.69,18 21.69,21.37 22.86,22.54 23.95,22.54 IC1.18
MCLR
  Top 0.406: ICSP.1 9.38,20.71 R18.1 9.31,19.9 9.84,19.37 11.75,19.37 13.65,21.27 15.88,21.27 16.51,21.91 16.51,26.04 17.6,27.12 IC2.4
MS1-1  (via drill 0.5)
  Top 0.406: SJ1.1 58.42,4.45 59.69,5.71 59.69,23.5 v59.37,23.81
  Bottom 0.406: IC1.44 36.46,27.62 38.73,27.62 40.01,26.35 48.58,26.35 49.53,25.4 50.16,25.4 50.8,26.04 51.44,26.04 52.07,25.4 54.61,25.4 55.24,24.77 55.24,24.13 55.88,23.5 59.05,23.5 v59.37,23.81
MS1-2
  Bottom 0.406: IC1.11 31.49,18.73 35.56,18.73 39.37,22.54 46.67,22.54 47.62,21.59 64.77,21.59 66.36,23.18 SJ2.1
MS2-1  (via drill 0.5)
  Top 0.406: M1.3 50.8,10.79 50.8,19.05 49.85,20 v49.85,26.35
  Bottom 0.406: IC1.43 36.27,29.21 38.1,29.21 40.32,26.99 49.21,26.99 v49.85,26.35
MS2-2
  Bottom 0.406: IC1.34 31.49,34.61 35.24,34.61 36.83,33.02 40.01,33.02 42.23,30.8 52.39,30.8 53.98,29.21 60.64,29.21 64.14,25.72 67.31,25.72 69.53,27.94 71.12,27.94 72.39,26.67 72.39,22.54 70.48,20.64 M2.3
MS3-1  (via drill 0.5)
  Top 0.406: M1.4 SJ1.3 58.42,10.16 58.42,22.54 56.52,24.45 v56.2,24.45
  Bottom 0.406: IC1.42 35.78,29.84 38.42,29.84 40.64,27.62 50.8,27.62 52.39,26.04 54.93,26.04 56.2,24.77 v56.2,24.45
MS3-2
  Bottom 0.406: IC1.35 31.99,33.97 34.92,33.97 36.51,32.38 39.69,32.38 41.91,30.16 52.07,30.16 53.66,28.57 60.33,28.57 63.82,25.08 67.63,25.08 69.85,27.3 70.8,27.3 71.75,26.35 71.75,22.86 70.8,21.91 69.53,21.91 68.58,20.95 68.58,19.68 | 68.58,19.68 M2.4 | 68.58,19.68 SJ2.3
MS13-1
  Top 0.406: M1.2 55.24,4.45 SJ1.2
MS13-2
  Top 0.406: M2.2 69.53,23.18 SJ2.2
N$1
  Bottom 0.406: R2.1 2.67,8.57 HCSPEED.1
PWM  (via drill 0.5)
  Top 0.406: v33.66,28.57 33.66,30.8 v29.84,34.61
  Bottom 0.406: IC1.41 33.66,28.85 v33.66,28.57 | v29.84,34.61 28.89,35.56 28.89,36.83 37.2,45.13 Q1.1
PWM-OD
  Bottom 0.813: Q1.3 39.37,39.5 PWM.3
PWM-RES
  Bottom 0.813: Q1.2 42.18,45.13 R22.2
PWRLED
  Top 0.406: R14.2 61.49,33.55 PWR.A
RA+/SO
  Bottom 0.406: IC1.30 25.44,32.7 24.45,32.7 19.37,27.62 19.37,18.41 22.23,15.56 22.23,13.97 22.86,13.34 22.86,10.79 21.59,9.53 21.59,8.89 20.95,8.26 ST4.6
RA-1A
  Top 1.93: JP1.4 79.38,20.64 80.64,19.37 80.64,16.51 81.6,15.56 M2.12
RA-1B
  Bottom 1.93: JP1.1 M2.11
RA-2A
  Bottom 1.93: JP1.2 79.69,15.56 82.23,18.1 M2.13
RA-2B
  Bottom 1.93: JP1.3 79.06,18.1 81.6,20.64 M2.14
RA-/!SS
  Bottom 0.406: IC1.33 26.93,34.61 23.5,34.61 17.46,28.57 17.46,14.92 16.51,13.97 16.51,12.7 17.14,12.06 ST4.3
RESET  (via drill 0.5)
  Top 0.406: v24.13,27.62 23.07,27.62 C9.2 | PROG.5 23.81,39.05 24.45,38.42 26.04,38.42 28.89,35.56 30.16,35.56 34.92,30.8 34.92,28.26 34.29,27.62 33.66,27.62 32.7,26.67 | R20.1 32.7,26.67 | 32.7,26.67 32.7,25.72 v33.66,24.77
  Bottom 0.406: v24.13,27.62 27.62,27.62 28.26,28.26 29.84,28.26 33.34,24.77 v33.66,24.77 33.66,24.49 IC1.4
RX  (via drill 0.5)
  Top 0.406: v29.21,26.67 29.21,29.21 25.72,32.7 24.34,32.7 R16.1
  Bottom 0.406: IC1.7 32.05,22.7 31.73,22.7 29.84,24.59 29.84,26.04 v29.21,26.67
RX(USB)
  Top 0.406: IC2.12 16.72,30.37 18.1,31.75 20,31.75 20.95,32.7 R16.2
STAT-SCLK  (via drill 0.5)
  Top 0.406: v36.2,22.86 35.88,22.86 35.24,23.5 35.24,26.35 35.56,26.67 35.56,31.11 30.16,36.51 v29.84,36.51 28.89,36.51 26.35,39.05 PROG.3 | v56.2,31.43 56.62,31.85 R13.1
  Bottom 0.406: IC1.3 36.2,23.08 v36.2,22.86 | v29.84,36.51 30.16,36.51 31.43,35.24 35.56,35.24 35.88,34.92 37.47,34.92 38.1,34.29 40.64,34.29 42.86,32.07 43.5,32.07 44.77,33.34 54.93,33.34 56.2,32.07 v56.2,31.43
STATLED
  Top 0.406: R13.2 55.78,33.55 STAT.A
STEP-1  (via drill 0.5)
  Top 0.406: v51.12,25.08 51.12,20.64 M1.7
  Bottom 0.406: v51.12,25.08 50.8,24.77 49.21,24.77 48.26,25.72 39.69,25.72 38.73,26.67 35.56,26.67 34.61,25.72 33.34,25.72 30.16,28.89 27.94,28.89 27.3,28.26 25.36,28.26 IC1.26
STEP-2  (via drill 0.5)
  Top 0.406: M2.7 69.85,10.48 64.14,16.19 64.14,22.23 v63.82,22.54
  Bottom 0.406: IC1.10 31.99,19.37 35.24,19.37 39.05,23.18 46.99,23.18 47.94,22.23 63.5,22.23 v63.82,22.54
SWITCH
  Bottom 3: D1.C 64.88,46.35 60.64,46.35 58.74,44.45 | 58.74,44.45 55.56,41.27 | 55.56,41.27 PWR-SW.COM | 55.56,41.27 PWR-SW.NO 58.74,41.53 58.74,44.45
TX  (via drill 0.5)
  Top 0.406: v27.94,26.67 28.26,26.99 28.26,29.21 26.35,31.11 R15.1
  Bottom 0.406: v27.94,26.67 27.94,26.99 28.57,27.62 29.53,27.62 33.34,23.81 33.34,23.67 IC1.5
TX(USB)
  Top 0.406: IC2.10 20.97,31.02 R15.2
USBLED
  Bottom 0.406: R19.1 48.51,32 USB.A
USBOSC1
  Top 0.406: IC2.2 20.21,25.82 20.64,25.4 20.64,23.5 20.32,23.18 19.43,23.18 X2.2 18.8,22.29 17.88,21.38 C8.1
USBOSC2
  Top 0.406: IC2.3 20.52,26.47 21.27,25.72 21.27,23.5 21.59,23.18 22.16,23.18 X2.1 23.07,22.26 C7.1
USBSTAT  (via drill 0.5)
  Top 0.406: v37.15,33.97 35.56,33.97 31.11,38.42 31.11,43.5 29.84,44.77 27.94,44.77 27.3,45.4 v24.13,45.4 | v15.24,28.26 14.76,27.77 IC2.16
  Bottom 0.406: v37.15,33.97 37.47,33.66 40.32,33.66 42.55,31.43 44.55,31.43 R19.2 | v24.13,45.4 23.81,45.4 21.91,43.5 21.91,34.92 v15.24,28.26
V+
  Top 1.016: IC3.2 19.93,45.82 C10.1 22.64,45.82 23.5,46.67 29.53,46.67 32.23,43.97 32.23,38.89 33.81,37.31 36.86,37.31 PWM.2
  Top 1.778: PWM.2 37.27,37.02 37.47,36.83 42.86,36.83
  Top 1.93: 44.77,2.54 44.77,1.91 M1.16 38.06,1.91 C4.+
  Top 2.184: C2.+ 82.55,26.04 M2.16 83.19,26.04 83.19,27.94 82.23,28.89 81.28,28.89
  Top 3: PWR-SW.NC 49.59,44.39 47.62,46.35 44.77,46.35 42.86,44.45 42.86,36.83 45.4,34.29 45.4,28.89 | 45.4,28.89 45.4,3.17 44.77,2.54 | 45.4,28.89 81.28,28.89 82.55,27.62
VBUS
  Top 0.406: D2.2 4.33,31.31 USB->.1
VIN
  Bottom 3: D1.A 73.23,42.82 J1.CENTRE
VPIC
  Top 0.406: R18.2 10.88,20.77 ICSP.2 10.88,23.41 10.48,23.81 8.57,23.81 8.26,23.5 8.26,22.64 | IC2.1 18.19,25.17 17.14,24.13 17.14,21.59 16.19,20.64 13.97,20.64 12.06,18.73 8.57,18.73 8.26,19.05 8.26,22.23 | 8.26,22.23 8.26,22.64 | D2.1 2.02,22.74 2.54,22.23 8.26,22.23 | C5.1 8.26,22.64
VUSB
  Top 0.406: IC2.17 10.02,27.12 8.47,28.68 C6.2

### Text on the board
tPlace: =8834 | =882x/498x | Jumpers: | 1 2 3
tNames: 12V
bNames: Designed By | Thomas Carpenter | (C) 2013-26 | AstroEQ | V4.8-SMD | RA
Reference: This board design is for AstroEQ boards which fit inside the enclosure on an EQ5 Mount. | The board uses some very tricky surface mount components and is not recommended for DIY. | It is a 2 Layer board designed to be sent for manufacture. The AstroEQ-SMD-Gerber.zip file contains the required gerber files. | I use iteadstudio.com 10cm x 5cm prototype service, selecting 1.2mm thick, HASL, 100% electrical check

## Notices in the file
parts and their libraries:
SparkFun: Licensing: CC v3.0 Share-Alike You are welcome to use this library for commercial purposes.
